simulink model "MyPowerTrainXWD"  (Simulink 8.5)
settings: Solver=ode1  SolverMode=SingleTasking  StartTime=0.0  StopTime=inf  FixedStep=0.0002  RelTol=1e-3
PreLoadFcn:
  | vehicle = 'Car'; if ~length(which('cmself')), cmenv; end
  | MyPowerTrainXWD_bus
InitFcn:
  | vehicle = 'Car'; if ~length(which('cmself')), cmenv; end
  | MyPowerTrainXWD_bus
undefined symbols (not defined in the file or in its folder): float
libraries: simulink x1

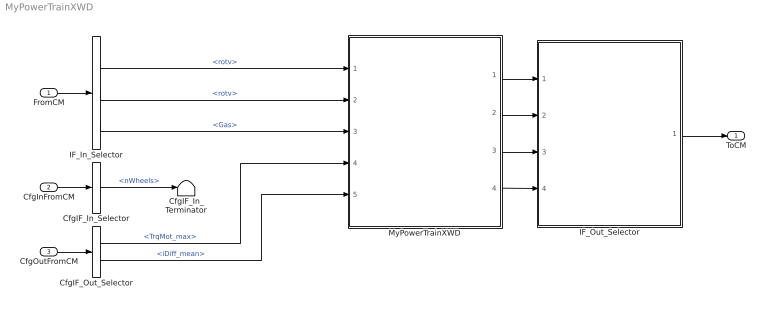
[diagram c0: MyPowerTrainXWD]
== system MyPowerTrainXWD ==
  FromCM : Inport  OutDataTypeStr=Bus: cmPowerTrainXWDIn
  CfgInFromCM : Inport  Port=2  OutDataTypeStr=Bus: cmPowerTrainXWDCfgIn
  CfgOutFromCM : Inport  Port=3  OutDataTypeStr=Bus: cmPowerTrainXWDCfgOut
  CfgIF_In_Selector : BusSelector  OutputSignals=nWheels
  CfgIF_In_Terminator : Terminator
  CfgIF_Out_Selector : BusSelector  OutputSignals=Motor.m0.TrqMot_max,DriveLine.iDiff_mean
  IF_In_Selector : BusSelector  OutputSignals=WheelIn.FL.rotv,WheelIn.FR.rotv,Gas
  IF_Out_Selector : Subsystem
  MyPowerTrainXWD : Subsystem
  ToCM : Outport  OutDataTypeStr=Bus: cmPowerTrainXWDOut
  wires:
  FromCM/1 -> IF_In_Selector/1
  IF_Out_Selector/1(ToCM) -> ToCM/1
  CfgInFromCM/1 -> CfgIF_In_Selector/1
  CfgIF_In_Selector/1 -> CfgIF_In_Terminator/1  "<nWheels>"
  CfgOutFromCM/1 -> CfgIF_Out_Selector/1
  MyPowerTrainXWD/1(PT.WFL.Trq_Drive) -> IF_Out_Selector/1(WheelOut.FL.Trq_Drive)
  MyPowerTrainXWD/2(PT.WFR.Trq_Drive) -> IF_Out_Selector/2(WheelOut.FR.Trq_Drive)
  MyPowerTrainXWD/3(PT.WFL.Trq_Supp2WC) -> IF_Out_Selector/3(WheelOut.FL.Trq_Supp2WC)
  MyPowerTrainXWD/4(PT.WFR.Trq_Supp2WC) -> IF_Out_Selector/4(WheelOut.FR.Trq_Supp2WC)
  IF_In_Selector/1 -> MyPowerTrainXWD/1(PT.WFL.rotv)  "<rotv>"
  IF_In_Selector/2 -> MyPowerTrainXWD/2(PT.WFR.rotv)  "<rotv>"
  CfgIF_Out_Selector/1 -> MyPowerTrainXWD/4(TrqMotor_Max)  "<TrqMot_max>"
  CfgIF_Out_Selector/2 -> MyPowerTrainXWD/5(iDiff_mean)  "<iDiff_mean>"
  IF_In_Selector/3 -> MyPowerTrainXWD/3(Gas)  "<Gas>"

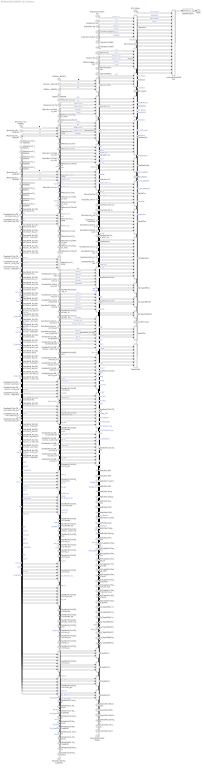
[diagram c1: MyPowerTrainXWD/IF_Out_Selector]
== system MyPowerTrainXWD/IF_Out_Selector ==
  WheelOut.FL.Trq_Drive : Inport
  WheelOut.FR.Trq_Drive : Inport  Port=2
  WheelOut.FL.Trq_Supp2WC : Inport  Port=3
  WheelOut.FR.Trq_Supp2WC : Inport  Port=4
  BCU_Status : Constant  Value=0
  BattHVOut : BusCreator  Inputs=7
  BattHVOut.AOC : Constant  Value=0
  BattHVOut.Current : Constant  Value=0
  BattHVOut.Energy : Constant  Value=0
  BattHVOut.Pwr_max : Constant  Value=0
  BattHVOut.SOC : Constant  Value=0
  BattHVOut.SOH : Constant  Value=0
  BattHVOut.Temp : Constant  Value=0
  BattLVOut : BusCreator  Inputs=7
  BattLVOut.AOC : Constant  Value=0
  BattLVOut.Current : Constant  Value=0
  BattLVOut.Energy : Constant  Value=0
  BattLVOut.Pwr_max : Constant  Value=0
  BattLVOut.SOC : Constant  Value=0
  BattLVOut.SOH : Constant  Value=0
  BattLVOut.Temp : Constant  Value=0
  ClutchOut : BusCreator  Inputs=6
  ClutchOut.Pos : Constant  Value=0
  ClutchOut.Trq_in : Constant  Value=0
  ClutchOut.Trq_out : Constant  Value=0
  ClutchOut.i_TrqIn2Out : Constant  Value=0
  ClutchOut.rotv_in : Constant  Value=0
  ClutchOut.rotv_out : Constant  Value=0
  DL_iDiff_mean : Constant  Value=0
  ECU_Status : Constant  Value=0
  EngineOut : BusCreator  Inputs=7
  EngineOut.Engine_on : Constant  Value=0
  EngineOut.FuelFlow : Constant  Value=0
  EngineOut.Trq : Constant  Value=0
  EngineOut.TrqDrag : Constant  Value=0
  EngineOut.TrqFull : Constant  Value=0
  EngineOut.TrqOpt : Constant  Value=0
  EngineOut.rotv : Constant  Value=0
  GearBoxM_Out : BusCreator
  GearBoxM_Out.GB_m{0..3} (4 alike) : BusCreator  Inputs=10
  GearBoxM_Out.GB_m0.Clutch : BusCreator  Inputs=6
  GearBoxM_Out.GB_m0.Clutch.Pos : Constant  Value=0
  GearBoxM_Out.GB_m0.Clutch.Trq_in : Constant  Value=0
  GearBoxM_Out.GB_m0.Clutch.Trq_out : Constant  Value=0
  GearBoxM_Out.GB_m0.Clutch.i_TrqIn2Out : Constant  Value=0
  GearBoxM_Out.GB_m0.Clutch.rotv_in : Constant  Value=0
  GearBoxM_Out.GB_m0.Clutch.rotv_out : Constant  Value=0
  GearBoxM_Out.GB_m0.Clutch_dis : BusCreator  Inputs=6
  GearBoxM_Out.GB_m0.Clutch_dis.Pos : Constant  Value=0
  GearBoxM_Out.GB_m0.Clutch_dis.Trq_in : Constant  Value=0
  GearBoxM_Out.GB_m0.Clutch_dis.Trq_out : Constant  Value=0
  GearBoxM_Out.GB_m0.Clutch_dis.i_TrqIn2Out : Constant  Value=0
  GearBoxM_Out.GB_m0.Clutch_dis.rotv_in : Constant  Value=0
  GearBoxM_Out.GB_m0.Clutch_dis.rotv_out : Constant  Value=0
  GearBoxM_Out.GB_m0.GearNo : Constant  Value=0
  GearBoxM_Out.GB_m0.GearNo_dis : Constant  Value=0
  GearBoxM_Out.GB_m0.Trq_DriveSrc_trg : Constant  Value=0
  GearBoxM_Out.GB_m0.Trq_in : Constant  Value=0
  GearBoxM_Out.GB_m0.Trq_out : Constant  Value=0
  GearBoxM_Out.GB_m0.i : Constant  Value=0
  GearBoxM_Out.GB_m0.rotv_in : Constant  Value=0
  GearBoxM_Out.GB_m0.rotv_out : Constant  Value=0
  GearBoxM_Out.GB_m1.Clutch : BusCreator  Inputs=6
  GearBoxM_Out.GB_m1.Clutch.Pos : Constant  Value=0
  GearBoxM_Out.GB_m1.Clutch.Trq_in : Constant  Value=0
  GearBoxM_Out.GB_m1.Clutch.Trq_out : Constant  Value=0
  GearBoxM_Out.GB_m1.Clutch.i_TrqIn2Out : Constant  Value=0
  GearBoxM_Out.GB_m1.Clutch.rotv_in : Constant  Value=0
  GearBoxM_Out.GB_m1.Clutch.rotv_out : Constant  Value=0
  GearBoxM_Out.GB_m1.Clutch_dis : BusCreator  Inputs=6
  GearBoxM_Out.GB_m1.Clutch_dis.Pos : Constant  Value=0
  GearBoxM_Out.GB_m1.Clutch_dis.Trq_in : Constant  Value=0
  GearBoxM_Out.GB_m1.Clutch_dis.Trq_out : Constant  Value=0
  GearBoxM_Out.GB_m1.Clutch_dis.i_TrqIn2Out : Constant  Value=0
  GearBoxM_Out.GB_m1.Clutch_dis.rotv_in : Constant  Value=0
  GearBoxM_Out.GB_m1.Clutch_dis.rotv_out : Constant  Value=0
  GearBoxM_Out.GB_m1.GearNo : Constant  Value=0
  GearBoxM_Out.GB_m1.GearNo_dis : Constant  Value=0
  GearBoxM_Out.GB_m1.Trq_DriveSrc_trg : Constant  Value=0
  GearBoxM_Out.GB_m1.Trq_in : Constant  Value=0
  GearBoxM_Out.GB_m1.Trq_out : Constant  Value=0
  GearBoxM_Out.GB_m1.i : Constant  Value=0
  GearBoxM_Out.GB_m1.rotv_in : Constant  Value=0
  GearBoxM_Out.GB_m1.rotv_out : Constant  Value=0
  GearBoxM_Out.GB_m2.Clutch : BusCreator  Inputs=6
  GearBoxM_Out.GB_m2.Clutch.Pos : Constant  Value=0
  GearBoxM_Out.GB_m2.Clutch.Trq_in : Constant  Value=0
  GearBoxM_Out.GB_m2.Clutch.Trq_out : Constant  Value=0
  GearBoxM_Out.GB_m2.Clutch.i_TrqIn2Out : Constant  Value=0
  GearBoxM_Out.GB_m2.Clutch.rotv_in : Constant  Value=0
  GearBoxM_Out.GB_m2.Clutch.rotv_out : Constant  Value=0
  GearBoxM_Out.GB_m2.Clutch_dis : BusCreator  Inputs=6
  GearBoxM_Out.GB_m2.Clutch_dis.Pos : Constant  Value=0
  GearBoxM_Out.GB_m2.Clutch_dis.Trq_in : Constant  Value=0
  GearBoxM_Out.GB_m2.Clutch_dis.Trq_out : Constant  Value=0
  GearBoxM_Out.GB_m2.Clutch_dis.i_TrqIn2Out : Constant  Value=0
  GearBoxM_Out.GB_m2.Clutch_dis.rotv_in : Constant  Value=0
  GearBoxM_Out.GB_m2.Clutch_dis.rotv_out : Constant  Value=0
  GearBoxM_Out.GB_m2.GearNo : Constant  Value=0
  GearBoxM_Out.GB_m2.GearNo_dis : Constant  Value=0
  GearBoxM_Out.GB_m2.Trq_DriveSrc_trg : Constant  Value=0
  GearBoxM_Out.GB_m2.Trq_in : Constant  Value=0
  GearBoxM_Out.GB_m2.Trq_out : Constant  Value=0
  GearBoxM_Out.GB_m2.i : Constant  Value=0
  GearBoxM_Out.GB_m2.rotv_in : Constant  Value=0
  GearBoxM_Out.GB_m2.rotv_out : Constant  Value=0
  GearBoxM_Out.GB_m3.Clutch : BusCreator  Inputs=6
  GearBoxM_Out.GB_m3.Clutch.Pos : Constant  Value=0
  GearBoxM_Out.GB_m3.Clutch.Trq_in : Constant  Value=0
  GearBoxM_Out.GB_m3.Clutch.Trq_out : Constant  Value=0
  GearBoxM_Out.GB_m3.Clutch.i_TrqIn2Out : Constant  Value=0
  GearBoxM_Out.GB_m3.Clutch.rotv_in : Constant  Value=0
  GearBoxM_Out.GB_m3.Clutch.rotv_out : Constant  Value=0
  GearBoxM_Out.GB_m3.Clutch_dis : BusCreator  Inputs=6
  GearBoxM_Out.GB_m3.Clutch_dis.Pos : Constant  Value=0
  GearBoxM_Out.GB_m3.Clutch_dis.Trq_in : Constant  Value=0
  GearBoxM_Out.GB_m3.Clutch_dis.Trq_out : Constant  Value=0
  GearBoxM_Out.GB_m3.Clutch_dis.i_TrqIn2Out : Constant  Value=0
  GearBoxM_Out.GB_m3.Clutch_dis.rotv_in : Constant  Value=0
  GearBoxM_Out.GB_m3.Clutch_dis.rotv_out : Constant  Value=0
  GearBoxM_Out.GB_m3.GearNo : Constant  Value=0
  GearBoxM_Out.GB_m3.GearNo_dis : Constant  Value=0
  GearBoxM_Out.GB_m3.Trq_DriveSrc_trg : Constant  Value=0
  GearBoxM_Out.GB_m3.Trq_in : Constant  Value=0
  GearBoxM_Out.GB_m3.Trq_out : Constant  Value=0
  GearBoxM_Out.GB_m3.i : Constant  Value=0
  GearBoxM_Out.GB_m3.rotv_in : Constant  Value=0
  GearBoxM_Out.GB_m3.rotv_out : Constant  Value=0
  GearBoxOut : BusCreator  Inputs=10
  GearBoxOut.Clutch : BusCreator  Inputs=6
  GearBoxOut.Clutch.Pos : Constant  Value=0
  GearBoxOut.Clutch.Trq_in : Constant  Value=0
  GearBoxOut.Clutch.Trq_out : Constant  Value=0
  GearBoxOut.Clutch.i_TrqIn2Out : Constant  Value=0
  GearBoxOut.Clutch.rotv_in : Constant  Value=0
  GearBoxOut.Clutch.rotv_out : Constant  Value=0
  GearBoxOut.Clutch_dis : BusCreator  Inputs=6
  GearBoxOut.Clutch_dis.Pos : Constant  Value=0
  GearBoxOut.Clutch_dis.Trq_in : Constant  Value=0
  GearBoxOut.Clutch_dis.Trq_out : Constant  Value=0
  GearBoxOut.Clutch_dis.i_TrqIn2Out : Constant  Value=0
  GearBoxOut.Clutch_dis.rotv_in : Constant  Value=0
  GearBoxOut.Clutch_dis.rotv_out : Constant  Value=0
  GearBoxOut.GearNo : Constant  Value=0
  GearBoxOut.GearNo_dis : Constant  Value=0
  GearBoxOut.Trq_DriveSrc_trg : Constant  Value=0
  GearBoxOut.Trq_in : Constant  Value=0
  GearBoxOut.Trq_out : Constant  Value=0
  GearBoxOut.i : Constant  Value=0
  GearBoxOut.rotv_in : Constant  Value=0
  GearBoxOut.rotv_out : Constant  Value=0
  ISGOut : BusCreator  Inputs=6
  ISGOut.PwrElec : Constant  Value=0
  ISGOut.Trq : Constant  Value=0
  ISGOut.TrqGen_max : Constant  Value=0
  ISGOut.TrqMot_max : Constant  Value=0
  ISGOut.i_M2W : BusCreator
  ISGOut.i_M2W.FL : Constant  Value=0
  ISGOut.i_M2W.FR : Constant  Value=0
  ISGOut.i_M2W.RL : Constant  Value=0
  ISGOut.i_M2W.RR : Constant  Value=0
  ISGOut.rotv : Constant  Value=0
  MCU_Status : Constant  Value=0
  MotorOut : BusCreator
  MotorOut.m{0..3} (4 alike) : BusCreator  Inputs=6
  MotorOut.m0.PwrElec : Constant  Value=0
  MotorOut.m0.Trq : Constant  Value=0
  MotorOut.m0.TrqGen_max : Constant  Value=0
  MotorOut.m0.TrqMot_max : Constant  Value=0
  MotorOut.m0.i_M2W : BusCreator
  MotorOut.m0.i_M2W.FL : Constant  Value=0
  MotorOut.m0.i_M2W.FR : Constant  Value=0
  MotorOut.m0.i_M2W.RL : Constant  Value=0
  MotorOut.m0.i_M2W.RR : Constant  Value=0
  MotorOut.m0.rotv : Constant  Value=0
  MotorOut.m1.PwrElec : Constant  Value=0
  MotorOut.m1.Trq : Constant  Value=0
  MotorOut.m1.TrqGen_max : Constant  Value=0
  MotorOut.m1.TrqMot_max : Constant  Value=0
  MotorOut.m1.i_M2W : BusCreator
  MotorOut.m1.i_M2W.FL : Constant  Value=0
  MotorOut.m1.i_M2W.FR : Constant  Value=0
  MotorOut.m1.i_M2W.RL : Constant  Value=0
  MotorOut.m1.i_M2W.RR : Constant  Value=0
  MotorOut.m1.rotv : Constant  Value=0
  MotorOut.m2.PwrElec : Constant  Value=0
  MotorOut.m2.Trq : Constant  Value=0
  MotorOut.m2.TrqGen_max : Constant  Value=0
  MotorOut.m2.TrqMot_max : Constant  Value=0
  MotorOut.m2.i_M2W : BusCreator
  MotorOut.m2.i_M2W.FL : Constant  Value=0
  MotorOut.m2.i_M2W.FR : Constant  Value=0
  MotorOut.m2.i_M2W.RL : Constant  Value=0
  MotorOut.m2.i_M2W.RR : Constant  Value=0
  MotorOut.m2.rotv : Constant  Value=0
  MotorOut.m3.PwrElec : Constant  Value=0
  MotorOut.m3.Trq : Constant  Value=0
  MotorOut.m3.TrqGen_max : Constant  Value=0
  MotorOut.m3.TrqMot_max : Constant  Value=0
  MotorOut.m3.i_M2W : BusCreator
  MotorOut.m3.i_M2W.FL : Constant  Value=0
  MotorOut.m3.i_M2W.FR : Constant  Value=0
  MotorOut.m3.i_M2W.RL : Constant  Value=0
  MotorOut.m3.i_M2W.RR : Constant  Value=0
  MotorOut.m3.rotv : Constant  Value=0
  PowerDelta : BusCreator  Inputs=7
  PowerDelta.Diffs : Constant  Value=0
  PowerDelta.Inert : Constant  Value=0
  PowerDelta.Inert_DL : Constant  Value=0
  PowerDelta.PlanetGear : Constant  Value=0
  PowerDelta.PowerSupply : Constant  Value=0
  PowerDelta.Shafts : Constant  Value=0
  PowerDelta.Spring_DL : Constant  Value=0
  PwrSupplyOut : BusCreator  Inputs=12
  PwrSupplyOut.Eta_HV1toHV2 : Constant  Value=0
  PwrSupplyOut.Eta_HV1toLV : Constant  Value=0
  PwrSupplyOut.Pwr_HV1 : Constant  Value=0
  PwrSupplyOut.Pwr_HV1toHV2 : Constant  Value=0
  PwrSupplyOut.Pwr_HV1toHV2_max : Constant  Value=0
  PwrSupplyOut.Pwr_HV1toLV : Constant  Value=0
  PwrSupplyOut.Pwr_HV1toLV_max : Constant  Value=0
  PwrSupplyOut.Pwr_HV2 : Constant  Value=0
  PwrSupplyOut.Pwr_LV : Constant  Value=0
  PwrSupplyOut.Voltage_HV1 : Constant  Value=0
  PwrSupplyOut.Voltage_HV2 : Constant  Value=0
  PwrSupplyOut.Voltage_LV : Constant  Value=0
  RateTransition : RateTransition  OutPortSampleTime=str2num(get_param(bdroot,'FixedStep'))
  TCU_Status : Constant  Value=0
  Trq_Supp2Bdy1 : BusCreator  Inputs=3
  Trq_Supp2Bdy1.rx : Constant  Value=0
  Trq_Supp2Bdy1.ry : Constant  Value=0
  Trq_Supp2Bdy1.rz : Constant  Value=0
  Trq_Supp2Bdy1B : BusCreator  Inputs=3
  Trq_Supp2Bdy1B.rx : Constant  Value=0
  Trq_Supp2Bdy1B.ry : Constant  Value=0
  Trq_Supp2Bdy1B.rz : Constant  Value=0
  Trq_Supp2BdyEng : BusCreator  Inputs=2
  Trq_Supp2BdyEng.rx : Constant  Value=0
  Trq_Supp2BdyEng.ry : Constant  Value=0
  WheelOut : BusCreator
  WheelOut.FL : BusCreator  Inputs=3
  WheelOut.FL.Inert_in : Constant  Value=0
  WheelOut.FR : BusCreator  Inputs=3
  WheelOut.FR.Inert_in : Constant  Value=0
  WheelOut.RL : BusCreator  Inputs=3
  WheelOut.RL.Inert_in : Constant  Value=0
  WheelOut.RL.Trq_Drive : Constant  Value=0
  WheelOut.RL.Trq_Supp2WC : Constant  Value=0
  WheelOut.RR : BusCreator  Inputs=3
  WheelOut.RR.Inert_in : Constant  Value=0
  WheelOut.RR.Trq_Drive : Constant  Value=0
  WheelOut.RR.Trq_Supp2WC : Constant  Value=0
  cmPowerTrainXWDOut : BusCreator  Inputs=19
  ToCM : Outport
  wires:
  RateTransition/1 -> ToCM/1
  cmPowerTrainXWDOut/1 -> RateTransition/1
  ECU_Status/1 -> cmPowerTrainXWDOut/1  "ECU_Status"
  EngineOut/1 -> cmPowerTrainXWDOut/2  "EngineOut"
  EngineOut.Engine_on/1 -> EngineOut/1  "Engine_on"
  EngineOut.rotv/1 -> EngineOut/2  "rotv"
  EngineOut.Trq/1 -> EngineOut/3  "Trq"
  EngineOut.TrqDrag/1 -> EngineOut/4  "TrqDrag"
  EngineOut.TrqFull/1 -> EngineOut/5  "TrqFull"
  EngineOut.TrqOpt/1 -> EngineOut/6  "TrqOpt"
  EngineOut.FuelFlow/1 -> EngineOut/7  "FuelFlow"
  MCU_Status/1 -> cmPowerTrainXWDOut/3  "MCU_Status"
  ISGOut/1 -> cmPowerTrainXWDOut/4  "ISGOut"
  ISGOut.rotv/1 -> ISGOut/1  "rotv"
  ISGOut.Trq/1 -> ISGOut/2  "Trq"
  ISGOut.TrqMot_max/1 -> ISGOut/3  "TrqMot_max"
  ISGOut.TrqGen_max/1 -> ISGOut/4  "TrqGen_max"
  ISGOut.PwrElec/1 -> ISGOut/5  "PwrElec"
  ISGOut.i_M2W/1 -> ISGOut/6  "i_M2W"
  ISGOut.i_M2W.FL/1 -> ISGOut.i_M2W/1  "FL"
  ISGOut.i_M2W.FR/1 -> ISGOut.i_M2W/2  "FR"
  ISGOut.i_M2W.RL/1 -> ISGOut.i_M2W/3  "RL"
  ISGOut.i_M2W.RR/1 -> ISGOut.i_M2W/4  "RR"
  MotorOut/1 -> cmPowerTrainXWDOut/5  "MotorOut"
  MotorOut.m0/1 -> MotorOut/1  "m0"
  MotorOut.m0.rotv/1 -> MotorOut.m0/1  "rotv"
  MotorOut.m0.Trq/1 -> MotorOut.m0/2  "Trq"
  MotorOut.m0.TrqMot_max/1 -> MotorOut.m0/3  "TrqMot_max"
  MotorOut.m0.TrqGen_max/1 -> MotorOut.m0/4  "TrqGen_max"
  MotorOut.m0.PwrElec/1 -> MotorOut.m0/5  "PwrElec"
  MotorOut.m0.i_M2W/1 -> MotorOut.m0/6  "i_M2W"
  MotorOut.m0.i_M2W.FL/1 -> MotorOut.m0.i_M2W/1  "FL"
  MotorOut.m0.i_M2W.FR/1 -> MotorOut.m0.i_M2W/2  "FR"
  MotorOut.m0.i_M2W.RL/1 -> MotorOut.m0.i_M2W/3  "RL"
  MotorOut.m0.i_M2W.RR/1 -> MotorOut.m0.i_M2W/4  "RR"
  MotorOut.m1/1 -> MotorOut/2  "m1"
  MotorOut.m1.rotv/1 -> MotorOut.m1/1  "rotv"
  MotorOut.m1.Trq/1 -> MotorOut.m1/2  "Trq"
  MotorOut.m1.TrqMot_max/1 -> MotorOut.m1/3  "TrqMot_max"
  MotorOut.m1.TrqGen_max/1 -> MotorOut.m1/4  "TrqGen_max"
  MotorOut.m1.PwrElec/1 -> MotorOut.m1/5  "PwrElec"
  MotorOut.m1.i_M2W/1 -> MotorOut.m1/6  "i_M2W"
  MotorOut.m1.i_M2W.FL/1 -> MotorOut.m1.i_M2W/1  "FL"
  MotorOut.m1.i_M2W.FR/1 -> MotorOut.m1.i_M2W/2  "FR"
  MotorOut.m1.i_M2W.RL/1 -> MotorOut.m1.i_M2W/3  "RL"
  MotorOut.m1.i_M2W.RR/1 -> MotorOut.m1.i_M2W/4  "RR"
  MotorOut.m2/1 -> MotorOut/3  "m2"
  MotorOut.m2.rotv/1 -> MotorOut.m2/1  "rotv"
  MotorOut.m2.Trq/1 -> MotorOut.m2/2  "Trq"
  MotorOut.m2.TrqMot_max/1 -> MotorOut.m2/3  "TrqMot_max"
  MotorOut.m2.TrqGen_max/1 -> MotorOut.m2/4  "TrqGen_max"
  MotorOut.m2.PwrElec/1 -> MotorOut.m2/5  "PwrElec"
  MotorOut.m2.i_M2W/1 -> MotorOut.m2/6  "i_M2W"
  MotorOut.m2.i_M2W.FL/1 -> MotorOut.m2.i_M2W/1  "FL"
  MotorOut.m2.i_M2W.FR/1 -> MotorOut.m2.i_M2W/2  "FR"
  MotorOut.m2.i_M2W.RL/1 -> MotorOut.m2.i_M2W/3  "RL"
  MotorOut.m2.i_M2W.RR/1 -> MotorOut.m2.i_M2W/4  "RR"
  MotorOut.m3/1 -> MotorOut/4  "m3"
  MotorOut.m3.rotv/1 -> MotorOut.m3/1  "rotv"
  MotorOut.m3.Trq/1 -> MotorOut.m3/2  "Trq"
  MotorOut.m3.TrqMot_max/1 -> MotorOut.m3/3  "TrqMot_max"
  MotorOut.m3.TrqGen_max/1 -> MotorOut.m3/4  "TrqGen_max"
  MotorOut.m3.PwrElec/1 -> MotorOut.m3/5  "PwrElec"
  MotorOut.m3.i_M2W/1 -> MotorOut.m3/6  "i_M2W"
  MotorOut.m3.i_M2W.FL/1 -> MotorOut.m3.i_M2W/1  "FL"
  MotorOut.m3.i_M2W.FR/1 -> MotorOut.m3.i_M2W/2  "FR"
  MotorOut.m3.i_M2W.RL/1 -> MotorOut.m3.i_M2W/3  "RL"
  MotorOut.m3.i_M2W.RR/1 -> MotorOut.m3.i_M2W/4  "RR"
  TCU_Status/1 -> cmPowerTrainXWDOut/6  "TCU_Status"
  ClutchOut/1 -> cmPowerTrainXWDOut/7  "ClutchOut"
  ClutchOut.Pos/1 -> ClutchOut/1  "Pos"
  ClutchOut.rotv_in/1 -> ClutchOut/2  "rotv_in"
  ClutchOut.rotv_out/1 -> ClutchOut/3  "rotv_out"
  ClutchOut.Trq_in/1 -> ClutchOut/4  "Trq_in"
  ClutchOut.Trq_out/1 -> ClutchOut/5  "Trq_out"
  ClutchOut.i_TrqIn2Out/1 -> ClutchOut/6  "i_TrqIn2Out"
  GearBoxOut/1 -> cmPowerTrainXWDOut/8  "GearBoxOut"
  GearBoxOut.GearNo/1 -> GearBoxOut/1  "GearNo"
  GearBoxOut.GearNo_dis/1 -> GearBoxOut/2  "GearNo_dis"
  GearBoxOut.Trq_DriveSrc_trg/1 -> GearBoxOut/3  "Trq_DriveSrc_trg"
  GearBoxOut.i/1 -> GearBoxOut/4  "i"
  GearBoxOut.rotv_in/1 -> GearBoxOut/5  "rotv_in"
  GearBoxOut.rotv_out/1 -> GearBoxOut/6  "rotv_out"
  GearBoxOut.Trq_in/1 -> GearBoxOut/7  "Trq_in"
  GearBoxOut.Trq_out/1 -> GearBoxOut/8  "Trq_out"
  GearBoxOut.Clutch/1 -> GearBoxOut/9  "Clutch"
  GearBoxOut.Clutch.Pos/1 -> GearBoxOut.Clutch/1  "Pos"
  GearBoxOut.Clutch.rotv_in/1 -> GearBoxOut.Clutch/2  "rotv_in"
  GearBoxOut.Clutch.rotv_out/1 -> GearBoxOut.Clutch/3  "rotv_out"
  GearBoxOut.Clutch.Trq_in/1 -> GearBoxOut.Clutch/4  "Trq_in"
  GearBoxOut.Clutch.Trq_out/1 -> GearBoxOut.Clutch/5  "Trq_out"
  GearBoxOut.Clutch.i_TrqIn2Out/1 -> GearBoxOut.Clutch/6  "i_TrqIn2Out"
  GearBoxOut.Clutch_dis/1 -> GearBoxOut/10  "Clutch_dis"
  GearBoxOut.Clutch_dis.Pos/1 -> GearBoxOut.Clutch_dis/1  "Pos"
  GearBoxOut.Clutch_dis.rotv_in/1 -> GearBoxOut.Clutch_dis/2  "rotv_in"
  GearBoxOut.Clutch_dis.rotv_out/1 -> GearBoxOut.Clutch_dis/3  "rotv_out"
  GearBoxOut.Clutch_dis.Trq_in/1 -> GearBoxOut.Clutch_dis/4  "Trq_in"
  GearBoxOut.Clutch_dis.Trq_out/1 -> GearBoxOut.Clutch_dis/5  "Trq_out"
  GearBoxOut.Clutch_dis.i_TrqIn2Out/1 -> GearBoxOut.Clutch_dis/6  "i_TrqIn2Out"
  GearBoxM_Out/1 -> cmPowerTrainXWDOut/9  "GearBoxM_Out"
  GearBoxM_Out.GB_m0/1 -> GearBoxM_Out/1  "GB_m0"
  GearBoxM_Out.GB_m0.GearNo/1 -> GearBoxM_Out.GB_m0/1  "GearNo"
  GearBoxM_Out.GB_m0.GearNo_dis/1 -> GearBoxM_Out.GB_m0/2  "GearNo_dis"
  GearBoxM_Out.GB_m0.Trq_DriveSrc_trg/1 -> GearBoxM_Out.GB_m0/3  "Trq_DriveSrc_trg"
  GearBoxM_Out.GB_m0.i/1 -> GearBoxM_Out.GB_m0/4  "i"
  GearBoxM_Out.GB_m0.rotv_in/1 -> GearBoxM_Out.GB_m0/5  "rotv_in"
  GearBoxM_Out.GB_m0.rotv_out/1 -> GearBoxM_Out.GB_m0/6  "rotv_out"
  GearBoxM_Out.GB_m0.Trq_in/1 -> GearBoxM_Out.GB_m0/7  "Trq_in"
  GearBoxM_Out.GB_m0.Trq_out/1 -> GearBoxM_Out.GB_m0/8  "Trq_out"
  GearBoxM_Out.GB_m0.Clutch/1 -> GearBoxM_Out.GB_m0/9  "Clutch"
  GearBoxM_Out.GB_m0.Clutch.Pos/1 -> GearBoxM_Out.GB_m0.Clutch/1  "Pos"
  GearBoxM_Out.GB_m0.Clutch.rotv_in/1 -> GearBoxM_Out.GB_m0.Clutch/2  "rotv_in"
  GearBoxM_Out.GB_m0.Clutch.rotv_out/1 -> GearBoxM_Out.GB_m0.Clutch/3  "rotv_out"
  GearBoxM_Out.GB_m0.Clutch.Trq_in/1 -> GearBoxM_Out.GB_m0.Clutch/4  "Trq_in"
  GearBoxM_Out.GB_m0.Clutch.Trq_out/1 -> GearBoxM_Out.GB_m0.Clutch/5  "Trq_out"
  GearBoxM_Out.GB_m0.Clutch.i_TrqIn2Out/1 -> GearBoxM_Out.GB_m0.Clutch/6  "i_TrqIn2Out"
  GearBoxM_Out.GB_m0.Clutch_dis/1 -> GearBoxM_Out.GB_m0/10  "Clutch_dis"
  GearBoxM_Out.GB_m0.Clutch_dis.Pos/1 -> GearBoxM_Out.GB_m0.Clutch_dis/1  "Pos"
  GearBoxM_Out.GB_m0.Clutch_dis.rotv_in/1 -> GearBoxM_Out.GB_m0.Clutch_dis/2  "rotv_in"
  GearBoxM_Out.GB_m0.Clutch_dis.rotv_out/1 -> GearBoxM_Out.GB_m0.Clutch_dis/3  "rotv_out"
  GearBoxM_Out.GB_m0.Clutch_dis.Trq_in/1 -> GearBoxM_Out.GB_m0.Clutch_dis/4  "Trq_in"
  GearBoxM_Out.GB_m0.Clutch_dis.Trq_out/1 -> GearBoxM_Out.GB_m0.Clutch_dis/5  "Trq_out"
  GearBoxM_Out.GB_m0.Clutch_dis.i_TrqIn2Out/1 -> GearBoxM_Out.GB_m0.Clutch_dis/6  "i_TrqIn2Out"
  GearBoxM_Out.GB_m1/1 -> GearBoxM_Out/2  "GB_m1"
  GearBoxM_Out.GB_m1.GearNo/1 -> GearBoxM_Out.GB_m1/1  "GearNo"
  GearBoxM_Out.GB_m1.GearNo_dis/1 -> GearBoxM_Out.GB_m1/2  "GearNo_dis"
  GearBoxM_Out.GB_m1.Trq_DriveSrc_trg/1 -> GearBoxM_Out.GB_m1/3  "Trq_DriveSrc_trg"
  GearBoxM_Out.GB_m1.i/1 -> GearBoxM_Out.GB_m1/4  "i"
  GearBoxM_Out.GB_m1.rotv_in/1 -> GearBoxM_Out.GB_m1/5  "rotv_in"
  GearBoxM_Out.GB_m1.rotv_out/1 -> GearBoxM_Out.GB_m1/6  "rotv_out"
  GearBoxM_Out.GB_m1.Trq_in/1 -> GearBoxM_Out.GB_m1/7  "Trq_in"
  GearBoxM_Out.GB_m1.Trq_out/1 -> GearBoxM_Out.GB_m1/8  "Trq_out"
  GearBoxM_Out.GB_m1.Clutch/1 -> GearBoxM_Out.GB_m1/9  "Clutch"
  GearBoxM_Out.GB_m1.Clutch.Pos/1 -> GearBoxM_Out.GB_m1.Clutch/1  "Pos"
  GearBoxM_Out.GB_m1.Clutch.rotv_in/1 -> GearBoxM_Out.GB_m1.Clutch/2  "rotv_in"
  GearBoxM_Out.GB_m1.Clutch.rotv_out/1 -> GearBoxM_Out.GB_m1.Clutch/3  "rotv_out"
  GearBoxM_Out.GB_m1.Clutch.Trq_in/1 -> GearBoxM_Out.GB_m1.Clutch/4  "Trq_in"
  GearBoxM_Out.GB_m1.Clutch.Trq_out/1 -> GearBoxM_Out.GB_m1.Clutch/5  "Trq_out"
  GearBoxM_Out.GB_m1.Clutch.i_TrqIn2Out/1 -> GearBoxM_Out.GB_m1.Clutch/6  "i_TrqIn2Out"
  GearBoxM_Out.GB_m1.Clutch_dis/1 -> GearBoxM_Out.GB_m1/10  "Clutch_dis"
  GearBoxM_Out.GB_m1.Clutch_dis.Pos/1 -> GearBoxM_Out.GB_m1.Clutch_dis/1  "Pos"
  GearBoxM_Out.GB_m1.Clutch_dis.rotv_in/1 -> GearBoxM_Out.GB_m1.Clutch_dis/2  "rotv_in"
  GearBoxM_Out.GB_m1.Clutch_dis.rotv_out/1 -> GearBoxM_Out.GB_m1.Clutch_dis/3  "rotv_out"
  GearBoxM_Out.GB_m1.Clutch_dis.Trq_in/1 -> GearBoxM_Out.GB_m1.Clutch_dis/4  "Trq_in"
  GearBoxM_Out.GB_m1.Clutch_dis.Trq_out/1 -> GearBoxM_Out.GB_m1.Clutch_dis/5  "Trq_out"
  GearBoxM_Out.GB_m1.Clutch_dis.i_TrqIn2Out/1 -> GearBoxM_Out.GB_m1.Clutch_dis/6  "i_TrqIn2Out"
  GearBoxM_Out.GB_m2/1 -> GearBoxM_Out/3  "GB_m2"
  GearBoxM_Out.GB_m2.GearNo/1 -> GearBoxM_Out.GB_m2/1  "GearNo"
  GearBoxM_Out.GB_m2.GearNo_dis/1 -> GearBoxM_Out.GB_m2/2  "GearNo_dis"
  GearBoxM_Out.GB_m2.Trq_DriveSrc_trg/1 -> GearBoxM_Out.GB_m2/3  "Trq_DriveSrc_trg"
  GearBoxM_Out.GB_m2.i/1 -> GearBoxM_Out.GB_m2/4  "i"
  GearBoxM_Out.GB_m2.rotv_in/1 -> GearBoxM_Out.GB_m2/5  "rotv_in"
  GearBoxM_Out.GB_m2.rotv_out/1 -> GearBoxM_Out.GB_m2/6  "rotv_out"
  GearBoxM_Out.GB_m2.Trq_in/1 -> GearBoxM_Out.GB_m2/7  "Trq_in"
  GearBoxM_Out.GB_m2.Trq_out/1 -> GearBoxM_Out.GB_m2/8  "Trq_out"
  GearBoxM_Out.GB_m2.Clutch/1 -> GearBoxM_Out.GB_m2/9  "Clutch"
  GearBoxM_Out.GB_m2.Clutch.Pos/1 -> GearBoxM_Out.GB_m2.Clutch/1  "Pos"
  GearBoxM_Out.GB_m2.Clutch.rotv_in/1 -> GearBoxM_Out.GB_m2.Clutch/2  "rotv_in"
  GearBoxM_Out.GB_m2.Clutch.rotv_out/1 -> GearBoxM_Out.GB_m2.Clutch/3  "rotv_out"
  GearBoxM_Out.GB_m2.Clutch.Trq_in/1 -> GearBoxM_Out.GB_m2.Clutch/4  "Trq_in"
  GearBoxM_Out.GB_m2.Clutch.Trq_out/1 -> GearBoxM_Out.GB_m2.Clutch/5  "Trq_out"
  GearBoxM_Out.GB_m2.Clutch.i_TrqIn2Out/1 -> GearBoxM_Out.GB_m2.Clutch/6  "i_TrqIn2Out"
  GearBoxM_Out.GB_m2.Clutch_dis/1 -> GearBoxM_Out.GB_m2/10  "Clutch_dis"
  GearBoxM_Out.GB_m2.Clutch_dis.Pos/1 -> GearBoxM_Out.GB_m2.Clutch_dis/1  "Pos"
  GearBoxM_Out.GB_m2.Clutch_dis.rotv_in/1 -> GearBoxM_Out.GB_m2.Clutch_dis/2  "rotv_in"
  GearBoxM_Out.GB_m2.Clutch_dis.rotv_out/1 -> GearBoxM_Out.GB_m2.Clutch_dis/3  "rotv_out"
  GearBoxM_Out.GB_m2.Clutch_dis.Trq_in/1 -> GearBoxM_Out.GB_m2.Clutch_dis/4  "Trq_in"
  GearBoxM_Out.GB_m2.Clutch_dis.Trq_out/1 -> GearBoxM_Out.GB_m2.Clutch_dis/5  "Trq_out"
  GearBoxM_Out.GB_m2.Clutch_dis.i_TrqIn2Out/1 -> GearBoxM_Out.GB_m2.Clutch_dis/6  "i_TrqIn2Out"
  GearBoxM_Out.GB_m3/1 -> GearBoxM_Out/4  "GB_m3"
  GearBoxM_Out.GB_m3.GearNo/1 -> GearBoxM_Out.GB_m3/1  "GearNo"
  GearBoxM_Out.GB_m3.GearNo_dis/1 -> GearBoxM_Out.GB_m3/2  "GearNo_dis"
  GearBoxM_Out.GB_m3.Trq_DriveSrc_trg/1 -> GearBoxM_Out.GB_m3/3  "Trq_DriveSrc_trg"
  GearBoxM_Out.GB_m3.i/1 -> GearBoxM_Out.GB_m3/4  "i"
  GearBoxM_Out.GB_m3.rotv_in/1 -> GearBoxM_Out.GB_m3/5  "rotv_in"
  GearBoxM_Out.GB_m3.rotv_out/1 -> GearBoxM_Out.GB_m3/6  "rotv_out"
  GearBoxM_Out.GB_m3.Trq_in/1 -> GearBoxM_Out.GB_m3/7  "Trq_in"
  GearBoxM_Out.GB_m3.Trq_out/1 -> GearBoxM_Out.GB_m3/8  "Trq_out"
  GearBoxM_Out.GB_m3.Clutch/1 -> GearBoxM_Out.GB_m3/9  "Clutch"
  GearBoxM_Out.GB_m3.Clutch.Pos/1 -> GearBoxM_Out.GB_m3.Clutch/1  "Pos"
  GearBoxM_Out.GB_m3.Clutch.rotv_in/1 -> GearBoxM_Out.GB_m3.Clutch/2  "rotv_in"
  GearBoxM_Out.GB_m3.Clutch.rotv_out/1 -> GearBoxM_Out.GB_m3.Clutch/3  "rotv_out"
  GearBoxM_Out.GB_m3.Clutch.Trq_in/1 -> GearBoxM_Out.GB_m3.Clutch/4  "Trq_in"
  GearBoxM_Out.GB_m3.Clutch.Trq_out/1 -> GearBoxM_Out.GB_m3.Clutch/5  "Trq_out"
  GearBoxM_Out.GB_m3.Clutch.i_TrqIn2Out/1 -> GearBoxM_Out.GB_m3.Clutch/6  "i_TrqIn2Out"
  GearBoxM_Out.GB_m3.Clutch_dis/1 -> GearBoxM_Out.GB_m3/10  "Clutch_dis"
  GearBoxM_Out.GB_m3.Clutch_dis.Pos/1 -> GearBoxM_Out.GB_m3.Clutch_dis/1  "Pos"
  GearBoxM_Out.GB_m3.Clutch_dis.rotv_in/1 -> GearBoxM_Out.GB_m3.Clutch_dis/2  "rotv_in"
  GearBoxM_Out.GB_m3.Clutch_dis.rotv_out/1 -> GearBoxM_Out.GB_m3.Clutch_dis/3  "rotv_out"
  GearBoxM_Out.GB_m3.Clutch_dis.Trq_in/1 -> GearBoxM_Out.GB_m3.Clutch_dis/4  "Trq_in"
  GearBoxM_Out.GB_m3.Clutch_dis.Trq_out/1 -> GearBoxM_Out.GB_m3.Clutch_dis/5  "Trq_out"
  GearBoxM_Out.GB_m3.Clutch_dis.i_TrqIn2Out/1 -> GearBoxM_Out.GB_m3.Clutch_dis/6  "i_TrqIn2Out"
  BCU_Status/1 -> cmPowerTrainXWDOut/10  "BCU_Status"
  BattLVOut/1 -> cmPowerTrainXWDOut/11  "BattLVOut"
  BattLVOut.SOC/1 -> BattLVOut/1  "SOC"
  BattLVOut.SOH/1 -> BattLVOut/2  "SOH"
  BattLVOut.Current/1 -> BattLVOut/3  "Current"
  BattLVOut.AOC/1 -> BattLVOut/4  "AOC"
  BattLVOut.Temp/1 -> BattLVOut/5  "Temp"
  BattLVOut.Energy/1 -> BattLVOut/6  "Energy"
  BattLVOut.Pwr_max/1 -> BattLVOut/7  "Pwr_max"
  BattHVOut/1 -> cmPowerTrainXWDOut/12  "BattHVOut"
  BattHVOut.SOC/1 -> BattHVOut/1  "SOC"
  BattHVOut.SOH/1 -> BattHVOut/2  "SOH"
  BattHVOut.Current/1 -> BattHVOut/3  "Current"
  BattHVOut.AOC/1 -> BattHVOut/4  "AOC"
  BattHVOut.Temp/1 -> BattHVOut/5  "Temp"
  BattHVOut.Energy/1 -> BattHVOut/6  "Energy"
  PwrSupplyOut/1 -> cmPowerTrainXWDOut/13  "PwrSupplyOut"
  PwrSupplyOut.Pwr_LV/1 -> PwrSupplyOut/1  "Pwr_LV"
  PwrSupplyOut.Pwr_HV1/1 -> PwrSupplyOut/2  "Pwr_HV1"
  PwrSupplyOut.Pwr_HV2/1 -> PwrSupplyOut/3  "Pwr_HV2"
  PwrSupplyOut.Voltage_LV/1 -> PwrSupplyOut/4  "Voltage_LV"
  PwrSupplyOut.Voltage_HV1/1 -> PwrSupplyOut/5  "Voltage_HV1"
  PwrSupplyOut.Voltage_HV2/1 -> PwrSupplyOut/6  "Voltage_HV2"
  PwrSupplyOut.Pwr_HV1toLV/1 -> PwrSupplyOut/7  "Pwr_HV1toLV"
  PwrSupplyOut.Pwr_HV1toHV2/1 -> PwrSupplyOut/8  "Pwr_HV1toHV2"
  PwrSupplyOut.Pwr_HV1toLV_max/1 -> PwrSupplyOut/9  "Pwr_HV1toLV_max"
  PwrSupplyOut.Pwr_HV1toHV2_max/1 -> PwrSupplyOut/10  "Pwr_HV1toHV2_max"
  PwrSupplyOut.Eta_HV1toLV/1 -> PwrSupplyOut/11  "Eta_HV1toLV"
  PwrSupplyOut.Eta_HV1toHV2/1 -> PwrSupplyOut/12  "Eta_HV1toHV2"
  Trq_Supp2Bdy1/1 -> cmPowerTrainXWDOut/14  "Trq_Supp2Bdy1"
  Trq_Supp2Bdy1.rx/1 -> Trq_Supp2Bdy1/1  "rx"
  Trq_Supp2Bdy1.ry/1 -> Trq_Supp2Bdy1/2  "ry"
  Trq_Supp2Bdy1.rz/1 -> Trq_Supp2Bdy1/3  "rz"
  Trq_Supp2Bdy1B/1 -> cmPowerTrainXWDOut/15  "Trq_Supp2Bdy1B"
  Trq_Supp2Bdy1B.rx/1 -> Trq_Supp2Bdy1B/1  "rx"
  Trq_Supp2Bdy1B.ry/1 -> Trq_Supp2Bdy1B/2  "ry"
  Trq_Supp2Bdy1B.rz/1 -> Trq_Supp2Bdy1B/3  "rz"
  Trq_Supp2BdyEng/1 -> cmPowerTrainXWDOut/16  "Trq_Supp2BdyEng"
  Trq_Supp2BdyEng.rx/1 -> Trq_Supp2BdyEng/1  "rx"
  Trq_Supp2BdyEng.ry/1 -> Trq_Supp2BdyEng/2  "ry"
  DL_iDiff_mean/1 -> cmPowerTrainXWDOut/17  "DL_iDiff_mean"
  WheelOut/1 -> cmPowerTrainXWDOut/18  "WheelOut"
  WheelOut.FL/1 -> WheelOut/1  "FL"
  WheelOut.FL.Inert_in/1 -> WheelOut.FL/1  "Inert_in"
  WheelOut.FR/1 -> WheelOut/2  "FR"
  WheelOut.FR.Inert_in/1 -> WheelOut.FR/1  "Inert_in"
  WheelOut.RL/1 -> WheelOut/3  "RL"
  WheelOut.RL.Inert_in/1 -> WheelOut.RL/1  "Inert_in"
  WheelOut.RL.Trq_Drive/1 -> WheelOut.RL/2  "Trq_Drive"
  WheelOut.RR/1 -> WheelOut/4  "RR"
  WheelOut.RR.Inert_in/1 -> WheelOut.RR/1  "Inert_in"
  WheelOut.RR.Trq_Drive/1 -> WheelOut.RR/2  "Trq_Drive"
  PowerDelta/1 -> cmPowerTrainXWDOut/19  "PowerDelta"
  PowerDelta.PlanetGear/1 -> PowerDelta/1  "PlanetGear"
  PowerDelta.Diffs/1 -> PowerDelta/2  "Diffs"
  PowerDelta.Shafts/1 -> PowerDelta/3  "Shafts"
  PowerDelta.Spring_DL/1 -> PowerDelta/4  "Spring_DL"
  PowerDelta.Inert_DL/1 -> PowerDelta/5  "Inert_DL"
  PowerDelta.Inert/1 -> PowerDelta/6  "Inert"
  PowerDelta.PowerSupply/1 -> PowerDelta/7  "PowerSupply"
  WheelOut.FL.Trq_Drive/1 -> WheelOut.FL/2  "Trq_Drive"
  WheelOut.FR.Trq_Drive/1 -> WheelOut.FR/2  "Trq_Drive"
  WheelOut.FL.Trq_Supp2WC/1 -> WheelOut.FL/3  "Trq_Supp2WC"
  WheelOut.FR.Trq_Supp2WC/1 -> WheelOut.FR/3  "Trq_Supp2WC"
  WheelOut.RL.Trq_Supp2WC/1 -> WheelOut.RL/3  "Trq_Supp2WC"
  WheelOut.RR.Trq_Supp2WC/1 -> WheelOut.RR/3  "Trq_Supp2WC"
  BattHVOut.Pwr_max/1 -> BattHVOut/7  "Pwr_max"

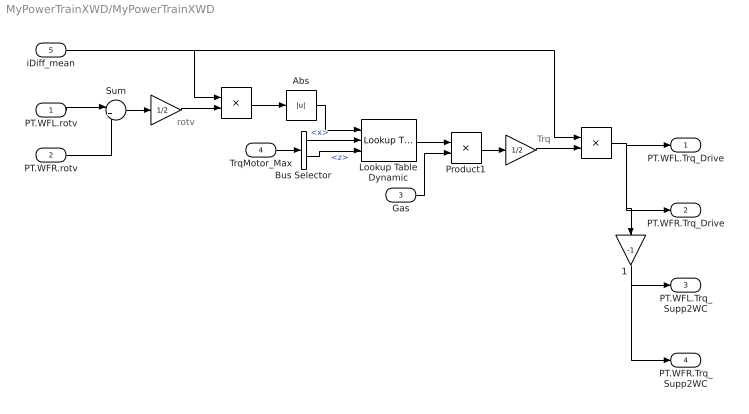
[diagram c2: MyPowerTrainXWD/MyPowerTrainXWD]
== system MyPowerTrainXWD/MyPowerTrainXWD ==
  note: Trq
  note: rotv
  PT.WFL.rotv : Inport
  PT.WFR.rotv : Inport  Port=2
  Gas : Inport  Port=3
  TrqMotor_Max : Inport  Port=4
  iDiff_mean : Inport  Port=5
  " " : Gain  Gain=1/2
  "  " : Gain  Gain=1/2
  "   " : Product
  "    " : Product
  "  1" : Gain  Gain=-1
  Abs : Abs
  Bus Selector : BusSelector  OutputSignals=x,z
  Lookup Table Dynamic : simulink/Lookup Tables/Lookup Table Dynamic  LookUpMeth=Interpolation-Use End Values  OutDataTypeStr=float('double')  OutputDataTypeScalingMode=Specify via dialog  OutDataType=float('double')  OutScaling=2^-10  DoSatur=off
  Product1 : Product
  Sum : Sum  Inputs=|++
  PT.WFL.Trq_Drive : Outport
  PT.WFR.Trq_Drive : Outport  Port=2
  PT.WFL.Trq_Supp2WC : Outport  Port=3
  PT.WFR.Trq_Supp2WC : Outport  Port=4
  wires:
  PT.WFL.rotv/1 -> Sum/1
  PT.WFR.rotv/1 -> Sum/2
  Sum/1 -> " "/1
  " "/1 -> "    "/2
  iDiff_mean/1 -> "    "/1, "   "/1
  "    "/1 -> Abs/1
  TrqMotor_Max/1 -> Bus Selector/1
  Bus Selector/1 -> Lookup Table Dynamic/2  "<x>"
  Bus Selector/2 -> Lookup Table Dynamic/3  "<z>"
  Abs/1 -> Lookup Table Dynamic/1
  Lookup Table Dynamic/1 -> Product1/1
  Gas/1 -> Product1/2
  Product1/1 -> "  "/1
  "  "/1 -> "   "/2
  "   "/1 -> PT.WFR.Trq_Drive/1, "  1"/1, PT.WFL.Trq_Drive/1
  "  1"/1 -> PT.WFR.Trq_Supp2WC/1, PT.WFL.Trq_Supp2WC/1
